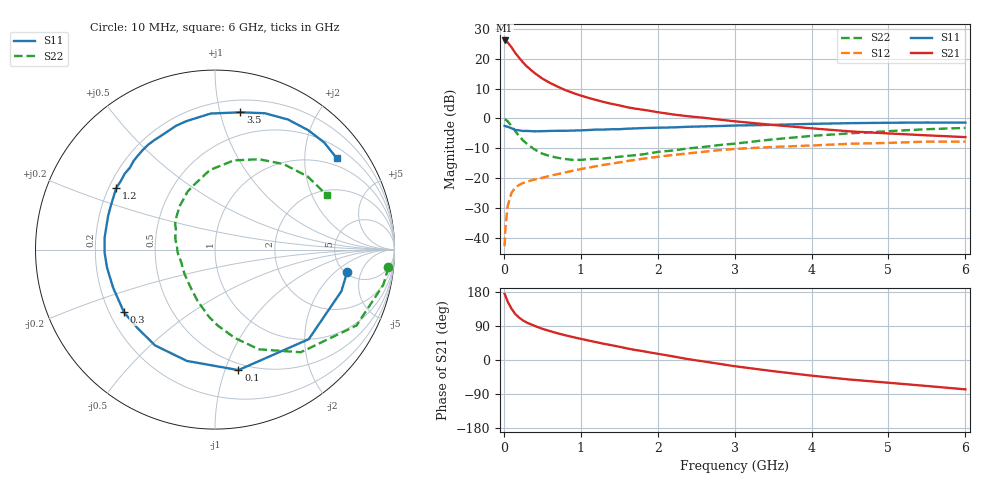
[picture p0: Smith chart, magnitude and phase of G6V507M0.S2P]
! SIEMENS Small Signal Semiconductors
! BFG193
! Si NPN RF Bipolar Junction Transistor in SOT223
! VCE = 0.5 V  IC = 7 mA
! Common Emitter S-Parameters:  August  1996
# GHz  S  MA  R  50
!  f  S11  S21  S12  S22
! GHz  MAG  ANG  MAG  ANG  MAG  ANG  MAG  ANG
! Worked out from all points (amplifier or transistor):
!   36 points, 10 MHz to 6 GHz, reference 50 ohm
!   highest |S21| = 26.1 dB at 10 MHz (marker M1)
!   |S21| within 3 dB of that: start of sweep to 118.3 MHz
!   unconditionally stable (mu >= 1): 888.9 MHz to 5.03 GHz; 5.717 GHz to end of sweep
!   at 250 MHz: K = 0.45, MSG = 20.2 dB, |S12| = -21.7 dB
!   at 1.4 GHz: K = 1.11, MAG = 8.0 dB, |S12| = -15.2 dB
!   at 6 GHz: K = 1.01, MAG = 0.2 dB, |S12| = -7.8 dB
!   S11 on the Smith chart (normalised r, x): 10 MHz: 5.26, -2.90; 100 MHz: 0.44, -1.11; 300 MHz: 0.26, -0.29; 1.2 GHz: 0.23, +0.27; 3.5 GHz: 0.30, +1.16; 6 GHz: 0.77, +2.81
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0.01  0.7471 -9.4  20.23 174.4  0.0072 88.6  0.9714 -5.8
0.02  0.7414 -18.2  20.1 169.8  0.0144 81.1  0.9582 -11.8
0.05  0.7224 -43.7  18.7 153.8  0.0338 68.8  0.8947 -28.2
0.1  0.6839 -79.0  15.55 135.4  0.0567 54.9  0.7456 -50.1
0.15  0.6398 -104.2  12.43 120.9  0.0692 45.5  0.6067 -66.3
0.2  0.6297 -122.1  10.32 111.7  0.0769 40.6  0.505 -77.3
0.25  0.6145 -135.0  8.634 104.2  0.0824 37.2  0.4255 -87.6
0.3  0.6158 -145.4  7.412 98.6  0.0867 36.2  0.3749 -95.3
0.4  0.606 -159.6  5.749 90.0  0.0944 34.6  0.3007 -109.0
0.5  0.6099 -170.5  4.653 82.4  0.1007 34.3  0.256 -120.9
0.6  0.6155 -178.5  3.927 76.3  0.1091 34.7  0.2325 -130.9
0.8  0.6186 168.2  2.976 65.2  0.1242 34.6  0.208 -149.7
0.9  0.6245 162.4  2.665 60.4  0.1328 34.5  0.2013 -157.7
1.1  0.6374 152.5  2.204 51.4  0.1489 33.9  0.2065 -171.7
1.2  0.6488 148.1  2.034 47.1  0.1577 33.4  0.2098 -178.2
1.7  0.6779 129.2  1.46 26.7  0.2006 27.2  0.2404 155.5
2.2  0.7053 113.5  1.163 9.5  0.2433 18.3  0.2892 136.6
2.8  0.7438 96.6  0.954 -10.1  0.2931 6.3  0.3566 115.6
3.5  0.778 79.5  0.776 -29.4  0.3318 -9.9  0.4443 93.7
4.5  0.831 60.7  0.605 -51.6  0.3751 -28.3  0.5605 63.9
5.5  0.8522 44.4  0.519 -68.6  0.4078 -50.1  0.6576 38.3
6  0.8482 36.9  0.485 -77.5  0.407 -62.6  0.6922 26.1
